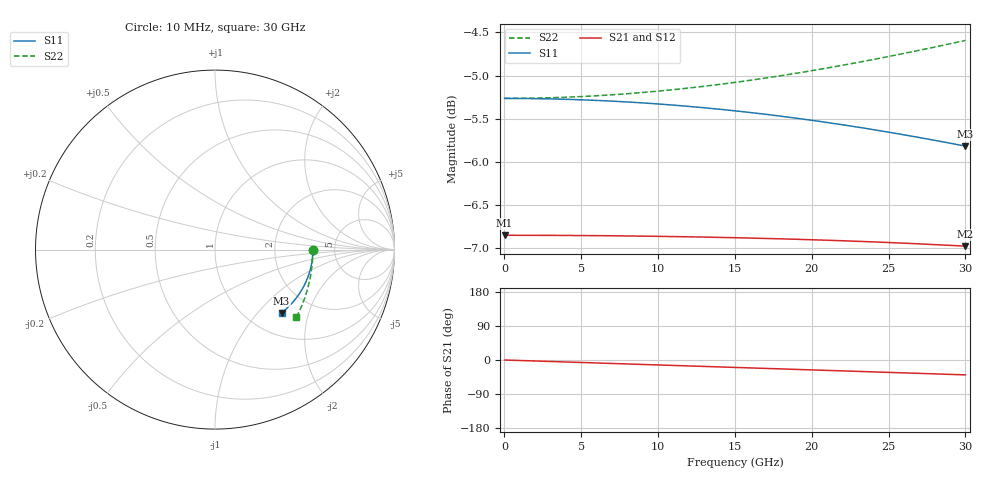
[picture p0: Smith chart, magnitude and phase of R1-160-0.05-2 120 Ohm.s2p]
!version-1
!date-04.2022
# GHz S RI R 50
!Freq ReS11 ImS11 ReS21 ImS21 ReS12 ImS12 ReS22 ImS22
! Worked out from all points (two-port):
!   601 points, 10 MHz to 30 GHz, reference 50 ohm
!   highest |S21| = -6.85 dB at 10 MHz (marker M1); lowest = -7.0 dB at 30 GHz (marker M2)
!   |S21| within 3 dB of the highest: start of sweep to end of sweep
!   lowest |S11| = -5.8 dB at 30 GHz (marker M3), VSWR 3.10, Z = 70.8 - j67.8 ohm
!   |S11| at or under -10 dB: nowhere
!   |S22| runs from -5.3 to -4.6 dB; largest |S21 - S12| = 1.4e-15
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0.01  0.5455 -0.000131  0.4545 -0.000103  0.4545 -0.000103  0.5455 -0.000131
0.16  0.5454 -0.00209  0.4545 -0.00164  0.4545 -0.00164  0.5455 -0.00209
2.51  0.5442 -0.0328  0.4538 -0.0258  0.4538 -0.0258  0.5448 -0.0328
3.76  0.5427 -0.0491  0.4528 -0.0386  0.4528 -0.0386  0.544 -0.0492
5.01  0.5405 -0.0654  0.4515 -0.0514  0.4515 -0.0514  0.5429 -0.0655
6.26  0.5377 -0.0815  0.4498 -0.0641  0.4498 -0.0641  0.5414 -0.0817
7.51  0.5343 -0.0976  0.4476 -0.0768  0.4476 -0.0768  0.5396 -0.098
8.76  0.5303 -0.1136  0.4452 -0.0894  0.4452 -0.0894  0.5375 -0.1142
10.01  0.5257 -0.1295  0.4423 -0.102  0.4423 -0.102  0.5351 -0.1303
11.26  0.5205 -0.1453  0.4391 -0.1144  0.4391 -0.1144  0.5324 -0.1464
12.51  0.5146 -0.1609  0.4355 -0.1268  0.4355 -0.1268  0.5293 -0.1625
13.76  0.5082 -0.1763  0.4315 -0.1391  0.4315 -0.1391  0.5259 -0.1784
15.01  0.5011 -0.1915  0.4271 -0.1512  0.4271 -0.1512  0.5223 -0.1943
16.26  0.4935 -0.2066  0.4224 -0.1632  0.4224 -0.1632  0.5182 -0.2101
17.51  0.4852 -0.2214  0.4173 -0.1751  0.4173 -0.1751  0.5139 -0.2258
20.01  0.4669 -0.2503  0.406 -0.1984  0.406 -0.1984  0.5043 -0.2569
22.51  0.4462 -0.2781  0.3932 -0.221  0.3932 -0.221  0.4935 -0.2875
25.01  0.4232 -0.3046  0.3791 -0.2428  0.3791 -0.2428  0.4814 -0.3176
26.41  0.4094 -0.3188  0.3705 -0.2547  0.3705 -0.2547  0.4742 -0.3342
27.81  0.3948 -0.3326  0.3616 -0.2662  0.3616 -0.2662  0.4665 -0.3506
29.81  0.3727 -0.3514  0.348 -0.2822  0.348 -0.2822  0.4549 -0.3737
30  0.3706 -0.3531  0.3467 -0.2837  0.3467 -0.2837  0.4538 -0.3759
